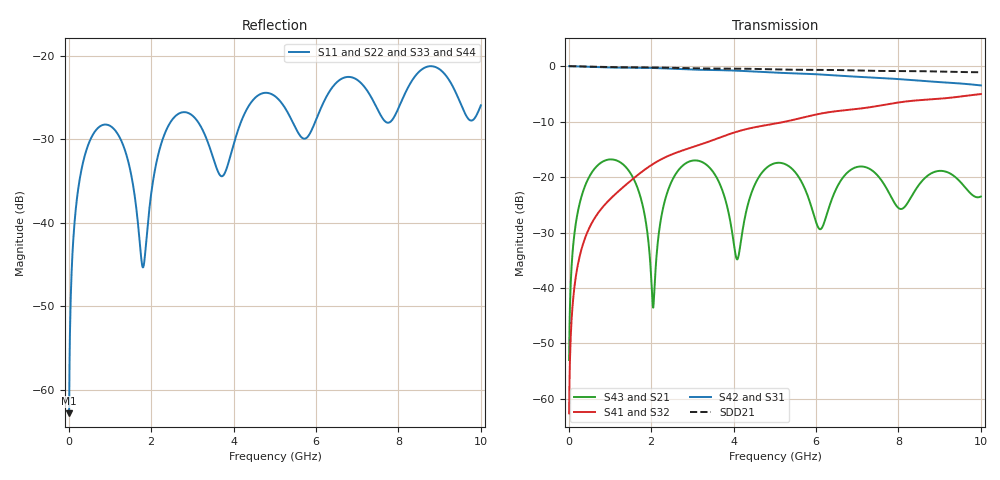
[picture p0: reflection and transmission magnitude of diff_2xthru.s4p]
# HZ S RI R 50
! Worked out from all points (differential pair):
!   1000 points, 10 MHz to 10 GHz, reference 50 ohm
!   strongest paths, dB at 10 MHz, 2.51 GHz, 5.01 GHz, 7.51 GHz, 10 GHz:
!     S42: 0.0, -0.5, -1.2, -2.1, -3.5
!     S31: 0.0, -0.5, -1.2, -2.1, -3.5
!     S41: -62.6, -15.9, -10.4, -7.2, -5.0
!     S32: -62.6, -15.9, -10.4, -7.2, -5.0
!     S43: -53.0, -20.6, -17.5, -19.8, -23.5
!     S21: -53.0, -20.6, -17.5, -19.8, -23.5
!   taken as a pair (ports 2,1 in; 4,3 out), SDD21 dB: 0.0, -0.3, -0.6, -0.9, -1.1
!   lowest |S11| = -62.8 dB at 10 MHz (marker M1), VSWR 1.00, Z = 50 + j0.0724 ohm
!   |S11| at or under -10 dB: start of sweep to end of sweep
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1e7  2.31e-05 0.000724  7.89e-05 0.00224  0.9996 -0.0153  1.67e-06 -0.000742
     7.89e-05 0.00224  2.31e-05 0.000724  1.67e-06 -0.000742  0.9996 -0.0153
     0.9996 -0.0153  1.67e-06 -0.000742  2.31e-05 0.000724  7.89e-05 0.00224
     1.67e-06 -0.000742  0.9996 -0.0153  7.89e-05 0.00224  2.31e-05 0.000724
7.7e8  0.037 0.00802  0.1243 0.0497  0.3804 -0.9009  -0.0485 -0.0144
       0.1243 0.0497  0.037 0.00802  -0.0485 -0.0144  0.3804 -0.9009
       0.3804 -0.9009  -0.0485 -0.0144  0.037 0.00802  0.1243 0.0497
       -0.0485 -0.0144  0.3804 -0.9009  0.1243 0.0497  0.037 0.00802
1.99e9  -0.00223 0.014  0.0075 -0.0124  -0.9571 -0.1175  -0.014 0.1264
        0.0075 -0.0124  -0.00223 0.014  -0.014 0.1264  -0.9571 -0.1175
        -0.9571 -0.1175  -0.014 0.1264  -0.00223 0.014  0.0075 -0.0124
        -0.014 0.1264  -0.9571 -0.1175  0.0075 -0.0124  -0.00223 0.014
4.1e9  0.000949 0.0353  0.0182 0.0018  0.9087 0.0445  0.00879 -0.2578
       0.0182 0.0018  0.000949 0.0353  0.00879 -0.2578  0.9087 0.0445
       0.9087 0.0445  0.00879 -0.2578  0.000949 0.0353  0.0182 0.0018
       0.00879 -0.2578  0.9087 0.0445  0.0182 0.0018  0.000949 0.0353
6.04e9  -0.0127 0.0417  0.0344 -0.0105  -0.8234 -0.1868  -0.0768 0.3609
        0.0344 -0.0105  -0.0127 0.0417  -0.0768 0.3609  -0.8234 -0.1868
        -0.8234 -0.1868  -0.0768 0.3609  -0.0127 0.0417  0.0344 -0.0105
        -0.0768 0.3609  -0.8234 -0.1868  0.0344 -0.0105  -0.0127 0.0417
8.17e9  0.00463 0.0599  0.054 0.00972  0.7525 0.0655  0.0322 -0.4787
        0.054 0.00972  0.00463 0.0599  0.0322 -0.4787  0.7525 0.0655
        0.7525 0.0655  0.0322 -0.4787  0.00463 0.0599  0.054 0.00972
        0.0322 -0.4787  0.7525 0.0655  0.054 0.00972  0.00463 0.0599
1e10  -0.0231 0.0448  0.0666 0.00446  -0.6188 -0.258  -0.2064 0.5209
      0.0666 0.00446  -0.0231 0.0448  -0.2064 0.5209  -0.6188 -0.258
      -0.6188 -0.258  -0.2064 0.5209  -0.0231 0.0448  0.0666 0.00446
      -0.2064 0.5209  -0.6188 -0.258  0.0666 0.00446  -0.0231 0.0448
